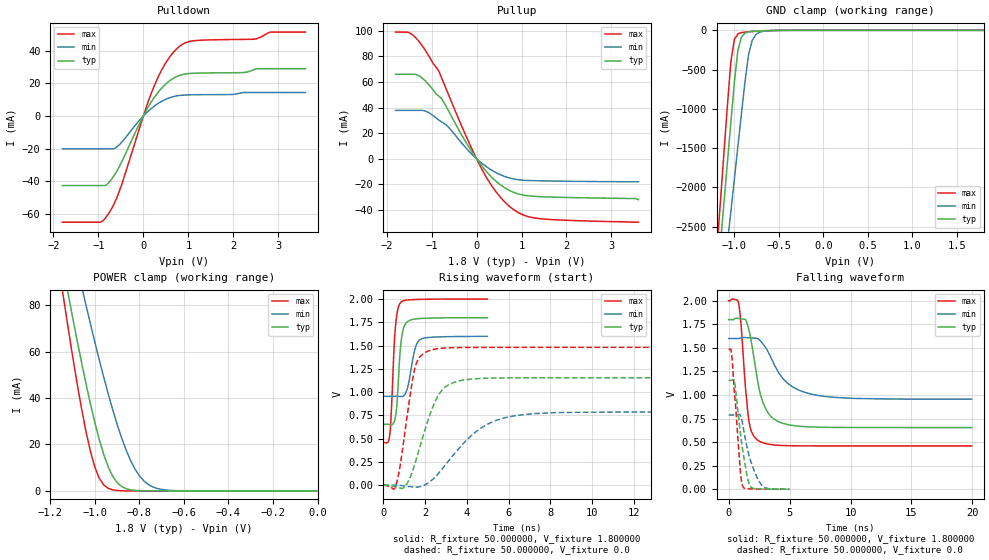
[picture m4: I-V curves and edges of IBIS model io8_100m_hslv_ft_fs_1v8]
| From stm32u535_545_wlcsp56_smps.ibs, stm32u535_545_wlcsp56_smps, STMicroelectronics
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|   Model io8_100m_hslv_ft_fs_1v8
[Model]  io8_100m_hslv_ft_fs_1v8
Model_type I/O
Polarity   Non-Inverting
Enable   Active-Low
Vinl =   0.540000V
Vinh =   1.260000V
Vmeas =  0.900000V
Cref =   50.000000pF
Rref =   100.000000M
Vref =   0.0V
C_comp   3.235100pF   3.233200pF   3.282800pF
[Temperature Range]   25.000000   0.140000k   -40.000000
[Pullup Reference]   1.800000V   1.600000V   2.000000V
[Pulldown Reference]   0.0V   0.0V   0.0V
[POWER Clamp Reference]   1.800000V   1.600000V   2.000000V
[GND Clamp Reference]   0.0V   0.0V   0.0V
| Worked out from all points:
|   slope of the pulldown table from 0 to 0.27 V, typ, clamps not added: 21.7 ohm
|   slope of the pullup table from 0 to 0.27 V, typ, clamps not added: 22.6 ohm
|   GND clamp passes 1 mA (typ) near -0.51 V on its own axis
|   POWER clamp passes 1 mA (typ) near -0.86 V on its own axis
|   rising waveform, R_fixture 50.000000, V_fixture 1.800000: 20-80 % time 212ps typ, 327ps min, 198ps max; typ from 0.654 V to 1.8 V
|   rising waveform, R_fixture 50.000000, V_fixture 0.0: 20-80 % time 1.03ns typ, 2.04ns min, 582ps max; typ from 0 V to 1.16 V
|   falling waveform, R_fixture 50.000000, V_fixture 1.800000: 20-80 % time 1.09ns typ, 2.1ns min, 568ps max; typ from 1.8 V to 0.654 V
|   falling waveform, R_fixture 50.000000, V_fixture 0.0: 20-80 % time 708ps typ, 989ps min, 510ps max; typ from 1.16 V to 0 V
[Pulldown]
|Voltage   I(typ)   I(min)   I(max)
-1.8V     -42.74mA   -20.21mA   -65.25mA
-960mV    -42.74mA   -20.21mA   -65.25mA
-780mV    -41.3mA    -20.21mA   -60.25mA
-540mV    -31.39mA   -17.82mA   -46.65mA
0V        -10fA      -600fA     10fA
240mV     11.28mA    6.002mA    18.38mA
480mV     19.18mA    10.02mA    31.83mA
780mV     24.67mA    12.5mA     42.21mA
1.14V     26.24mA    12.99mA    46.23mA
2.46V     28.42mA    14.39mA    47.14mA
2.82V     29mA       14.39mA    51.49mA
3.6V      29mA       14.39mA    51.49mA
[Pullup]
|Voltage   I(typ)   I(min)   I(max)
-1.8V     66.02mA    37.77mA    98.95mA
-1.44V    66.02mA    37.77mA    97.32mA
-1.14V    60.87mA    37.28mA    84.78mA
-840mV    48.93mA    30.23mA    68.56mA
-660mV    39.81mA    25.95mA    53.26mA
-300mV    16.72mA    11mA       23.08mA
120mV     -5.749mA   -3.603mA   -8.316mA
420mV     -17.18mA   -10.64mA   -25.23mA
780mV     -25.61mA   -15.48mA   -38.6mA
1.08V     -28.66mA   -16.9mA    -44.47mA
1.38V     -29.58mA   -17.26mA   -46.72mA
3.6V      -32mA      -18mA      -49.6mA
[GND_clamp]
|Voltage   I(typ)   I(min)   I(max)
-1.8V     -9.707A    -9.942A    -9.774A
-1.2V     -3.309A    -4.006A    -2.864A
-1.16V    -2.777A    -3.584A    -2.239A
-1.12V    -2.246A    -3.162A    -1.614A
-1.04V    -1.186A    -2.319A    -408.6mA
-1V       -663.9mA   -1.898A    -117.8mA
-960mV    -254mA     -1.478A    -45.14mA
-920mV    -86.03mA   -1.06A     -28.58mA
-840mV    -19.12mA   -308.9mA   -18.74mA
-800mV    -13.39mA   -130.8mA   -15.31mA
-720mV    -7.948mA   -25.37mA   -9.381mA
1.8V      0A         14.95nA    0A
[POWER_clamp]
|Voltage   I(typ)   I(min)   I(max)
-1.8V     470.8mA    433.7mA    554.6mA
-1.14V    95.25mA    122.7mA    82.82mA
-1.12V    84.97mA    114mA      70.27mA
-1.06V    55.51mA    88.42mA    35.67mA
-1.04V    46.34mA    80.15mA    25.76mA
-1V       29.51mA    64.13mA    10.3mA
-940mV    10.39mA    41.86mA    1.109mA
-900mV    3.624mA    28.77mA    182.8uA
-840mV    490.7uA    13.24mA    11.35uA
-800mV    116.8uA    6.532mA    1.77uA
-740mV    13.2uA     1.723mA    109.2nA
0V        0A         18.72nA    0A
[Ramp]
| variable   typ   min   max
dV/dt_r  0.69306/1.02378n   0.47204/2.03342n   0.88872/0.58146n
dV/dt_f  0.68761/1.08629n   0.38671/2.09301n   0.92481/0.56701n
R_load = 50.000000
[Rising Waveform]
R_fixture= 50.000000
V_fixture= 1.800000
V_fixture_min= 1.600000
V_fixture_max= 2.000000
|time   V(typ)   V(min)   V(max)
0s        654.1mV    955.5mV    458.8mV
310.3ps   653.2mV    955.6mV    550.1mV
370.4ps   651.2mV    955.8mV    747.2mV
550.6ps   707.7mV    956mV      1.629V
650.7ps   879.7mV    955.9mV    1.84V
810.8ps   1.458V     953.3mV    1.958V
1.061ns   1.735V     987.6mV    1.987V
1.512ns   1.786V     1.461V     1.995V
1.762ns   1.791V     1.564V     1.997V
4.985ns   1.8V       1.6V       2V
[Rising Waveform]
R_fixture= 50.000000
V_fixture= 0.0
V_fixture_min= 0.0
V_fixture_max= 0.0
|time   V(typ)   V(min)   V(max)
0s        -120.5uV   -24.73uV   -132.9uV
600.6ps   -17.04mV   -53.09uV   -901.2uV
1.041ns   -10.81mV   -9.087mV   586mV
1.522ns   239.3mV    -19.39mV   1.267V
2.242ns   764.6mV    40.38mV    1.45V
2.763ns   1.008V     159.9mV    1.471V
3.363ns   1.104V     327.7mV    1.478V
4.805ns   1.148V     631.8mV    1.481V
6.206ns   1.154V     742.9mV    1.481V
19.94ns   1.155V     786.9mV    1.481V
[Falling Waveform]
R_fixture= 50.000000
V_fixture= 1.800000
V_fixture_min= 1.600000
V_fixture_max= 2.000000
|time   V(typ)   V(min)   V(max)
0s        1.8V       1.6V       2V
800.8ps   1.812V     1.599V     1.984V
1.001ns   1.808V     1.607V     1.77V
1.361ns   1.802V     1.609V     1.105V
1.642ns   1.701V     1.607V     742.9mV
2.482ns   1.077V     1.59V      512.1mV
3.604ns   755.5mV    1.36V      471.3mV
4.885ns   684.3mV    1.119V     461.5mV
6.607ns   661.5mV    1.015V     459.2mV
19.94ns   654.1mV    955.5mV    458.8mV
[Falling Waveform]
R_fixture= 50.000000
V_fixture= 0.0
V_fixture_min= 0.0
V_fixture_max= 0.0
|time   V(typ)   V(min)   V(max)
0s        1.155V     786.9mV    1.481V
160.2ps   1.155V     786.9mV    1.486V
240.2ps   1.155V     786.9mV    1.434V
490.5ps   1.133V     787mV      998.9mV
971ps     583.4mV    781.2mV    174.7mV
1.171ns   398mV      672.9mV    25.66mV
1.512ns   139.1mV    442.2mV    4.306mV
1.712ns   47.02mV    339.1mV    2.982mV
2.673ns   2.336mV    49.1mV     744.6uV
4.985ns   -120.5uV   -24.73uV   -132.9uV
